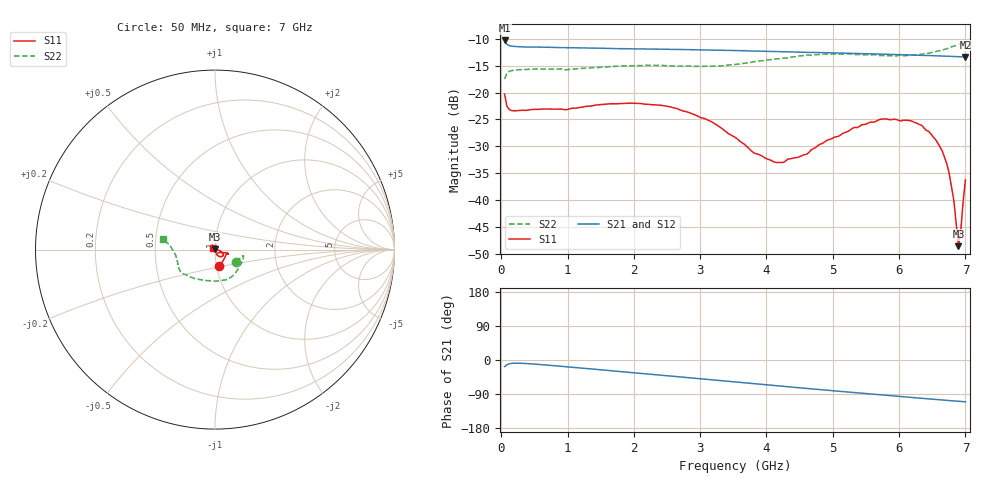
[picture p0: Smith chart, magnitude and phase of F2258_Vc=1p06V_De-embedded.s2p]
! Integrated Device Technology
! Corporate Headquarters
! 6024 Silver Creek Valley Road
! San Jose, CA 95138  USA
! Phone:  1-408-284-8200
! Toll Free:  1-800-223-1366
! Webpage:  http://www.idt.com/
! Timing and RF Division
! 515 Groton Road, Suite 102
! Westford, MA 01886-6024
! Device:  F2258
! Description: Voltage Variable RF Attenuator
! Frequency:  50.0 -  6000.00 MHz
! Package:  3x3 mm Thin QFN Plastic Package: 16 pin
! Ports:  2 RF, 2 DC
!  Pin  1  = NC
!  Pin  2  = NC
!  Pin  3  = RF2  = Port 2
!  Pin  4  = GND
!  Pin  5  = Vdd
!  Pin  6  = NC
!  Pin  7  = VCTRL
!  Pin  8  = NC
!  Pin  9  = GND
!  Pin 10  = RF1  = Port 1
!  Pin 11  = NC
!  Pin 12  = NC
!  Pin 13  = NC
!  Pin 14  = NC
!  Pin 15  = NC
!  Pin 16  = NC
! Vcntrl:  1.060 Volts
! Vdd:  +3.300 Volts
! Current:  1.161 mA
! Data:  The device was measured on a the F2258 evaluation board which has
!  individual transmission lines to the RF pins.  Data was collected
!  using a calibrated network analyzer.  The evaluation board was
!  de-embedded using a TRL calibration technique.
!  The reference plane is the edge of the package pin.
! Misc:  SN 10
!  Action Tracker AT0285
! Date Measured:  2014-12-10
! Date:  2016-01-13  MJV
! Note:
!  Integrated Device Technology supplies this data as a sample of measured
!  data at the package pin for this product.  Your particular data for this
!  product may vary.
!  Data was taken at 25 degrees C.
!  Integrated Device Technology reserves the right to change this data at anytime.
!Freq_(GHz)  S11M_(dB)  S11P_(deg)  S21M_(dB)  S21P_(deg)  S12M_(dB)  S12P_(deg)  S22M_(dB)  S22P_(deg)
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# GHz S dB R 50
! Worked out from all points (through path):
!   201 points, 50 MHz to 7 GHz, reference 50 ohm
!   highest |S21| = -10.33 dB at 50 MHz (marker M1); lowest = -13.4 dB at 7 GHz (marker M2)
!   group delay of S21, straight-line fit = 42.7 ps
!   lowest |S11| = -48.5 dB at 6.896 GHz (marker M3), VSWR 1.01, Z = 50.1 + j0.365 ohm
!   |S11| at or under -10 dB: start of sweep to end of sweep
!   |S22| runs from -17.5 to -10.5 dB; largest |S21 - S12| = 0.0014
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0.05  -20.31 -75.7  -10.33 -17.3  -10.30 -17.3  -17.47 -30.1
0.08475  -22.56 -49.2  -11.05 -12.3  -11.02 -12.2  -16.43 -16.7
0.15425  -23.35 -27.2  -11.38 -9.0  -11.36 -9.0  -15.93 -12.3
1.2315  -22.70 -18.2  -11.72 -21.7  -11.71 -21.7  -15.51 -39.6
2.37825  -22.35 -16.8  -11.95 -39.6  -11.97 -39.5  -14.94 -69.6
3.07325  -24.87 -18.0  -12.08 -50.7  -12.09 -50.7  -15.12 -92.9
3.525  -28.31 -25.0  -12.19 -58.0  -12.20 -58.0  -14.79 -111.0
3.803  -31.16 -37.8  -12.29 -62.5  -12.29 -62.5  -14.29 -121.6
4.1505  -33.01 -56.8  -12.39 -68.0  -12.38 -68.0  -13.74 -132.1
4.60225  -31.50 -73.0  -12.54 -75.0  -12.55 -74.9  -13.05 -142.5
4.7065  -30.42 -70.7  -12.54 -76.6  -12.57 -76.6  -13.03 -144.4
5.332  -26.46 -54.4  -12.74 -86.1  -12.78 -86.0  -12.94 -153.6
5.85325  -25.03 -39.4  -12.91 -93.8  -12.92 -93.8  -13.16 -163.6
6.33975  -26.08 -26.9  -13.09 -101.1  -13.11 -101.1  -12.88 -175.8
6.54825  -28.71 -20.4  -13.16 -104.1  -13.19 -104.1  -12.40 178.7
6.6525  -30.89 -14.3  -13.23 -105.5  -13.25 -105.5  -12.10 175.9
6.75675  -35.13 -7.8  -13.29 -107.1  -13.31 -107.0  -11.68 173.0
6.82625  -40.10 2.9  -13.30 -107.9  -13.32 -107.9  -11.39 171.9
6.89575  -48.54 76.8  -13.34 -108.9  -13.35 -108.9  -11.04 170.3
6.9305  -45.62 123.4  -13.34 -109.4  -13.36 -109.4  -10.92 169.9
6.96525  -40.38 144.1  -13.37 -109.9  -13.40 -109.8  -10.75 169.1
7  -36.23 145.8  -13.39 -110.3  -13.42 -110.3  -10.54 168.3
